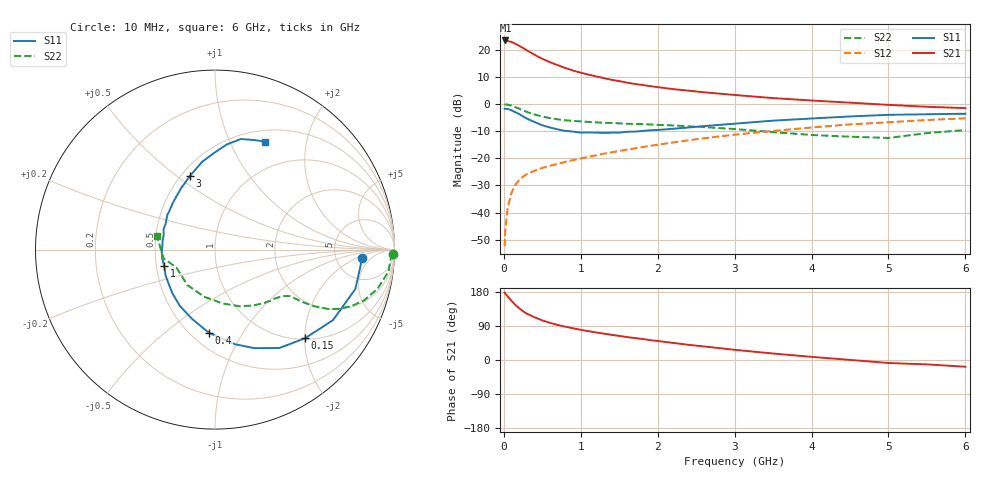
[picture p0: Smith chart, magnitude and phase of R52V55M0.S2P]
! SIEMENS Small Signal Semiconductors
! BFR183
! Si NPN RF Bipolar Junction Transistor in SOT23
! VCE = 2.5 V  IC = 5 mA
! Common Emitter S-Parameters:  May  1996
# GHz  S  MA  R  50
!  f  S11  S21  S12  S22
! GHz  MAG  ANG  MAG  ANG  MAG  ANG  MAG  ANG
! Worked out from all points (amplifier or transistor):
!   36 points, 10 MHz to 6 GHz, reference 50 ohm
!   highest |S21| = 23.4 dB at 20 MHz (marker M1)
!   |S21| within 3 dB of that: start of sweep to 261.5 MHz
!   unconditionally stable (mu >= 1): 1.007 GHz to 2.641 GHz
!   at 250 MHz: K = 0.42, MSG = 23.7 dB, |S12| = -26.7 dB
!   at 1.4 GHz: K = 1.06, MAG = 11.8 dB, |S12| = -17.8 dB
!   at 6 GHz: K = 0.89, MSG = 1.9 dB, |S12| = -5.2 dB
!   lowest NFmin = 1.15 dB at 450 MHz
!   S11 on the Smith chart (normalised r, x): 10 MHz: 9.31, -2.58; 150 MHz: 1.02, -2.00; 400 MHz: 0.61, -0.72; 1 GHz: 0.55, -0.11; 3 GHz: 0.55, +0.56; 6 GHz: 0.64, +1.37
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0.01  0.8188 -3.2  14.8 177.7  0.0024 87.7  0.9909 -1.4
0.02  0.8157 -6.6  14.87 174.8  0.0049 86.3  0.98 -2.9
0.05  0.8121 -15.7  14.57 167.7  0.0122 81.4  0.9751 -7.1
0.1  0.7658 -30.9  13.94 156.2  0.0233 75.1  0.932 -13.5
0.15  0.7039 -44.6  12.9 145.1  0.0325 68.3  0.8763 -18.9
0.2  0.6552 -56.8  11.82 136.5  0.0401 64.1  0.8209 -22.6
0.25  0.5904 -68.4  10.77 128.5  0.0461 60.7  0.764 -25.6
0.3  0.5392 -78.0  9.761 122.1  0.051 58.8  0.7144 -27.6
0.4  0.4653 -94.1  8.085 112.7  0.0593 56.3  0.641 -29.6
0.5  0.4059 -108.6  6.798 104.5  0.0665 54.9  0.5882 -30.6
0.6  0.3697 -121.9  5.913 98.0  0.0729 55.1  0.5497 -31.1
0.7  0.3413 -133.7  5.206 92.5  0.079 55.7  0.523 -31.4
0.8  0.3206 -143.8  4.61 87.8  0.0859 56.0  0.5023 -31.7
1  0.2976 -161.7  3.779 79.7  0.0993 57.0  0.4788 -32.6
1.1  0.2982 -170.0  3.489 76.2  0.1066 57.7  0.4687 -33.5
1.6  0.3083 158.3  2.483 60.5  0.1446 58.6  0.433 -38.6
2.2  0.3501 132.4  1.885 45.1  0.1959 56.7  0.4034 -47.8
3  0.4347 108.5  1.47 26.9  0.2728 50.5  0.3463 -65.9
3.5  0.4948 98.3  1.288 17.1  0.3198 45.0  0.3036 -81.8
4.5  0.5908 83.4  1.061 0.3  0.4219 33.0  0.2502 -128.1
5.5  0.6484 70.3  0.891 -11.6  0.5078 20.4  0.2914 -170.5
6  0.6633 65.1  0.841 -17.7  0.5472 12.3  0.3319 166.7
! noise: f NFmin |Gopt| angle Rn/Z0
0.45  1.15  0.25  40  0.26
0.9  1.2  0.25  93  0.22
1.8  1.95  0.32  170  0.13
